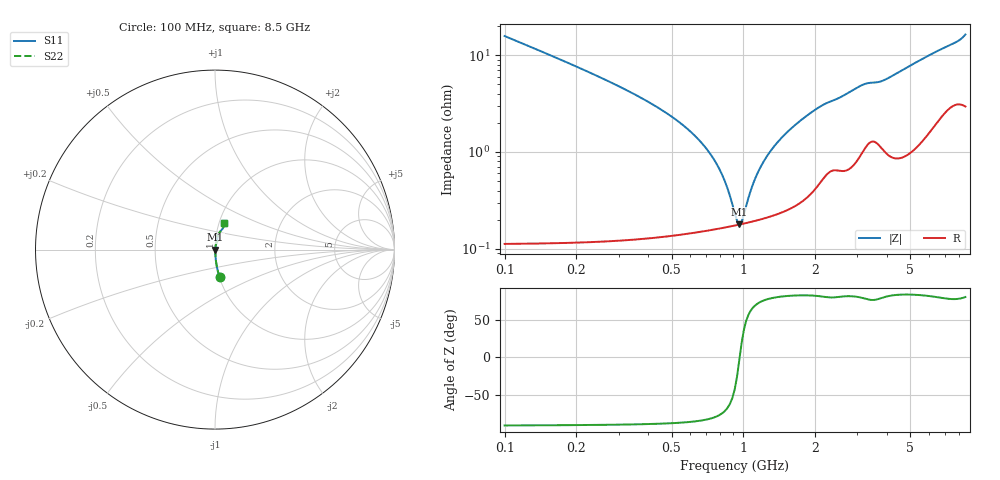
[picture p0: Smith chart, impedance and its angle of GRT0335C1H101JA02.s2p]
!Murata Part Number: GRT0335C1H101JA02
!These Parameters are Measured in Series Mode Connection
!Data Generated on Jun 19, 2026
!  o--ll--o
!Port1  Port2
!  o------o
!Operation Temp=25[degC], DC Bias Voltage=0[V]
!Freq. Start=100[MHz] Stop=9[GHz] 401[Steps]
# Hz S RI R 50
!Freq.(Hz) S11(Real) S11(Imag) S21(Real) S21(Imag) S12(Real) S12(Imag) S22(Real) S22(Imag)
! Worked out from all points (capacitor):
!   401 points, 100 MHz to 8.5 GHz, reference 50 ohm
!   read as one part in series: C = 100 pF near 142 MHz
!   lowest |Z| = 179 mohm at 961 MHz (marker M1)
!   series resonance near 964.3 MHz, so ESL is about 270 pH
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1e8  0.0252 -0.1533  0.9748 0.1533  0.9748 0.1533  0.0252 -0.1533
2.05e8  0.0066 -0.0735  0.9934 0.0735  0.9934 0.0735  0.0066 -0.0735
2.68e8  0.00417 -0.0544  0.9958 0.0544  0.9958 0.0544  0.00417 -0.0544
6.04e8  0.0017 -0.0159  0.9983 0.0159  0.9983 0.0159  0.0017 -0.0159
7.3e8  0.00165 -0.00924  0.9984 0.00924  0.9984 0.00924  0.00165 -0.00924
8.14e8  0.00167 -0.00558  0.9983 0.00558  0.9983 0.00558  0.00167 -0.00558
9.19e8  0.00174 -0.00158  0.9983 0.00158  0.9983 0.00158  0.00174 -0.00158
9.61e8  0.00178 -0.000112  0.9982 0.000112  0.9982 0.000112  0.00178 -0.000112
1.003e9  0.00182 0.00129  0.9982 -0.00129  0.9982 -0.00129  0.00182 0.00129
1.108e9  0.00195 0.00458  0.998 -0.00458  0.998 -0.00458  0.00195 0.00458
1.192e9  0.00207 0.00703  0.9979 -0.00703  0.9979 -0.00703  0.00207 0.00703
1.318e9  0.00229 0.0105  0.9977 -0.0105  0.9977 -0.0105  0.00229 0.0105
1.507e9  0.00271 0.0153  0.9973 -0.0153  0.9973 -0.0153  0.00271 0.0153
1.759e9  0.00352 0.0214  0.9965 -0.0214  0.9965 -0.0214  0.00352 0.0214
2.053e9  0.00527 0.0279  0.9947 -0.0279  0.9947 -0.0279  0.00527 0.0279
2.914e9  0.00929 0.0432  0.9907 -0.0432  0.9907 -0.0432  0.00929 0.0432
3.229e9  0.0131 0.0481  0.9869 -0.0481  0.9869 -0.0481  0.0131 0.0481
3.754e9  0.0137 0.051  0.9863 -0.051  0.9863 -0.051  0.0137 0.051
4.3e9  0.0123 0.0613  0.9877 -0.0613  0.9877 -0.0613  0.0123 0.0613
5.707e9  0.0215 0.0892  0.9785 -0.0892  0.9785 -0.0892  0.0215 0.0892
7.114e9  0.039 0.1122  0.961 -0.1122  0.961 -0.1122  0.039 0.1122
8.5e9  0.0517 0.148  0.9483 -0.148  0.9483 -0.148  0.0517 0.148
